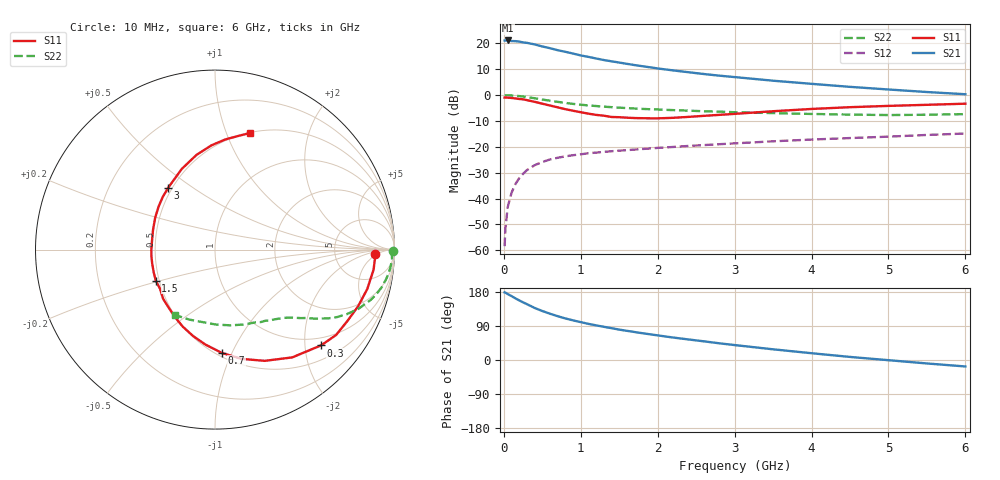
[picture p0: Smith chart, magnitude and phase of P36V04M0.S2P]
! SIEMENS Small Signal Semiconductors
! BFP181
! Si NPN RF Bipolar Junction Transistor in SOT143
! VCE = 6 V  IC = 4 mA
! Common Emitter S-Parameters:  March  1996
# GHz  S  MA  R  50
!  f  S11  S21  S12  S22
! GHz  MAG  ANG  MAG  ANG  MAG  ANG  MAG  ANG
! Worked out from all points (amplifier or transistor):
!   36 points, 10 MHz to 6 GHz, reference 50 ohm
!   highest |S21| = 21.1 dB at 50 MHz (marker M1)
!   |S21| within 3 dB of that: start of sweep to 601.3 MHz
!   unconditionally stable (mu >= 1): 1.953 GHz to end of sweep
!   at 250 MHz: K = 0.19, MSG = 25.4 dB, |S12| = -30.5 dB
!   at 1.4 GHz: K = 0.82, MSG = 17.4 dB, |S12| = -21.7 dB
!   at 6 GHz: K = 1.07, MAG = 6.0 dB, |S12| = -14.9 dB
!   S11 on the Smith chart (normalised r, x): 10 MHz: 17, -4; 300 MHz: 0.81, -2.36; 700 MHz: 0.53, -0.92; 1.5 GHz: 0.48, -0.19; 3 GHz: 0.48, +0.40; 6 GHz: 0.50, +1.22
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0.01  0.8912 -1.5  11.29 178.5  0.0012 83.7  0.9931 -0.5
0.02  0.8928 -2.9  11.31 177.8  0.0026 90.5  0.9855 -1.3
0.05  0.8906 -7.2  11.32 174.0  0.0068 89.0  0.9882 -3.3
0.15  0.8577 -21.6  10.99 162.7  0.019 77.2  0.9687 -9.6
0.2  0.8379 -28.4  10.77 157.3  0.0247 74.0  0.9531 -12.6
0.3  0.7962 -42.1  10.17 147.5  0.0354 67.2  0.9117 -17.9
0.4  0.7387 -54.4  9.499 137.4  0.044 61.6  0.865 -22.4
0.5  0.679 -65.9  8.667 129.3  0.0508 55.8  0.8178 -26.1
0.6  0.6267 -76.3  8.027 122.1  0.0568 52.1  0.7759 -29.0
0.7  0.5775 -86.1  7.34 115.6  0.0613 48.9  0.7376 -31.3
0.8  0.5321 -95.7  6.833 109.6  0.0653 46.3  0.7035 -33.1
0.9  0.4965 -104.3  6.318 104.6  0.0687 44.1  0.6733 -34.8
1.1  0.4361 -121.1  5.453 95.3  0.075 40.9  0.629 -37.3
1.3  0.3985 -136.5  4.741 87.6  0.0796 38.4  0.5955 -39.7
1.5  0.3725 -152.3  4.238 80.2  0.084 37.3  0.5692 -41.7
1.8  0.3563 -173.9  3.601 70.7  0.0904 35.6  0.5389 -44.8
2.2  0.3624 162.3  2.988 59.3  0.0991 33.6  0.5103 -49.6
3  0.4321 127.2  2.22 39.4  0.1163 30.3  0.4646 -60.7
3.5  0.486 112.4  1.89 28.2  0.1274 27.8  0.447 -69.1
4.5  0.5816 91.9  1.437 8.1  0.1473 21.8  0.4181 -89.0
5.5  0.6465 78.4  1.142 -9.1  0.1692 17.0  0.4157 -110.4
6  0.6796 73.1  1.035 -17.1  0.1803 13.7  0.4272 -121.5
